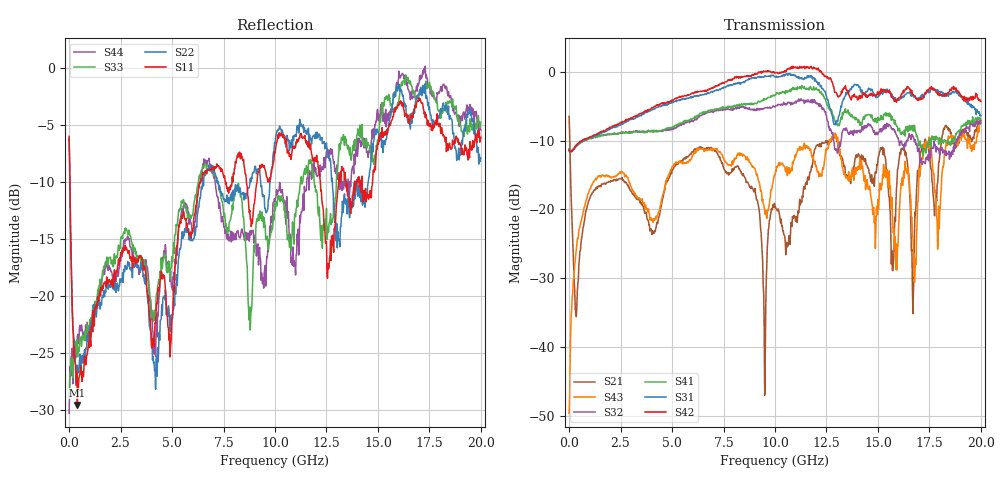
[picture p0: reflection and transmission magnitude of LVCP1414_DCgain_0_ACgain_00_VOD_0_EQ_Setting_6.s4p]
!Agilent Technologies,N5230A,MY46400459,A.07.50.48
!Agilent N5230A: A.07.50.48
!Date: Tuesday, April 17, 2012 18:35:17
!Correction: S11(Full 4 Port(1,2,3,4))
!S12(Full 4 Port(1,2,3,4))
!S13(Full 4 Port(1,2,3,4))
!S14(Full 4 Port(1,2,3,4))
!S21(Full 4 Port(1,2,3,4))
!S22(Full 4 Port(1,2,3,4))
!S23(Full 4 Port(1,2,3,4))
!S24(Full 4 Port(1,2,3,4))
!S31(Full 4 Port(1,2,3,4))
!S32(Full 4 Port(1,2,3,4))
!S33(Full 4 Port(1,2,3,4))
!S34(Full 4 Port(1,2,3,4))
!S41(Full 4 Port(1,2,3,4))
!S42(Full 4 Port(1,2,3,4))
!S43(Full 4 Port(1,2,3,4))
!S44(Full 4 Port(1,2,3,4))
!S4P File: Measurements: <S11,S12,S13,S14>,
!<S21,S22,S23,S24>,
!<S31,S32,S33,S34>,
!<S41,S42,S43,S44>:
# Hz S  dB  R 50
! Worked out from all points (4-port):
!   801 points, 300 kHz to 20 GHz, reference 50 ohm
!   strongest paths, dB at 300 kHz, 5 GHz, 10 GHz, 15 GHz, 20 GHz:
!     S42: -11.4, -4.1, -0.1, -3.0, -4.3
!     S31: -11.2, -4.4, -0.7, -3.6, -6.4
!     S41: -11.2, -8.0, -3.5, -6.6, -7.0
!     S32: -11.3, -8.3, -5.1, -9.0, -7.4
!     S43: -49.7, -13.8, -15.0, -18.5, -7.3
!     S21: -6.5, -14.3, -19.7, -12.7, -7.1
!   lowest |S11| = -29.5 dB at 400.3 MHz (marker M1), VSWR 1.07, Z = 53.2 + j1.4 ohm
!   |S11| at or under -10 dB: 37.56 MHz to 6.4 GHz (6.363 GHz wide, 198 % of centre); 8.614 GHz to 9.127 GHz (512.5 MHz wide, 5.78 % of centre); 12.2 GHz to 13.09 GHz (890.9 MHz wide, 7.04 % of centre)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
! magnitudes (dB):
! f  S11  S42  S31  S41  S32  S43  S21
! 300 kHz  -6.0  -11.4  -11.2  -11.2  -11.3  -49.7  -6.5
! 400.3 MHz  -29.5  -10.5  -10.5  -10.6  -10.6  -24.2  -31.8
! 9.5 GHz  -8.8  0.0  -0.6  -3.9  -5.2  -20.1  -47.0
! 10.05 GHz  -6.8  -0.1  -0.7  -3.3  -4.9  -14.5  -19.9
! 12.75 GHz  -14.7  -1.4  -6.1  -5.5  -8.8  -9.7  -10.0
! 16.8 GHz  -3.3  -3.5  -3.6  -8.3  -9.8  -29.2  -20.4
! 20 GHz  -6.1  -4.3  -6.4  -7.0  -7.4  -7.3  -7.1
